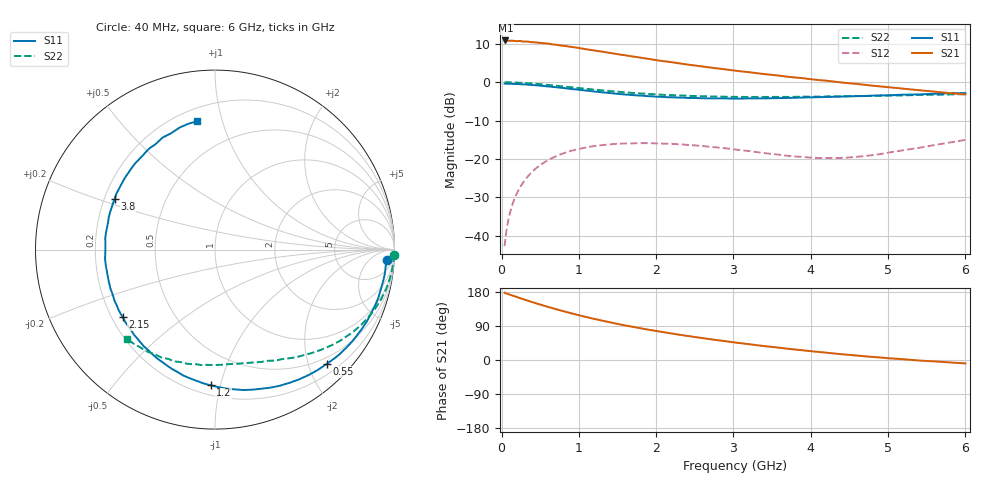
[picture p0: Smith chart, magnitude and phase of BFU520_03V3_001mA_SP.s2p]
! Filename:  P:\Prog\Test\Noise\ATS_data\Testdata_Net\03 Spar\BFU520_APG2013_37_A05_03p3V_001mA_SP_CM01_D.s2p
! Date/Time: Fri 26/Apr/2013 13:00:02
! BFU520_APG2013_37_A05_03p3V_1to20mA_SP_CM01_Bias1_R.s2p
! MDIF S-parameter v. bias file
! BFU520_APG2013_37_A05_03p3V_1to20mA_SP_CM01
! Date/time Tue Apr 23 14:11:50 2013
! bias mode 1
! bias variable = I_out
! VAR bias_var= 1
! VAR V_out= 3.3000
! VAR I_out= 0.9950
! VAR V_in= 0.7915
! VAR I_in= 0.0112
! Device data file deembeded for feedlines and parallel
! Original file: \03 Spar\BFU520_APG2013_37_A05_03p3V_001mA_SP_CM01_R.s2p
! Feed-files: PR047V01_250413_Feed1.s2p, PR047V01_250413_Feed2.s2p
! Parallel-file: PR047V01_250413_Par.s2p
# MHz S MA R 50
!  Freq-MHz  S11-mag  S11-arg  S21-mag  S21-arg  S12-mag  S12-arg  S22-mag  S22-arg
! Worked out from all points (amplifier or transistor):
!   98 points, 40 MHz to 6 GHz, reference 50 ohm
!   highest |S21| = 10.9 dB at 50 MHz (marker M1)
!   |S21| within 3 dB of that: start of sweep to 1.326 GHz
!   unconditionally stable (mu >= 1): 3.493 GHz to 5.423 GHz
!   at 300 MHz: K = 0.08, MSG = 18.1 dB, |S12| = -25.6 dB
!   at 1.6 GHz: K = 0.39, MSG = 11.5 dB, |S12| = -16.0 dB
!   at 6 GHz: K = 0.86, MSG = 5.9 dB, |S12| = -15.0 dB
!   S11 on the Smith chart (normalised r, x): 40 MHz: 16, -22; 550 MHz: 0.38, -2.32; 1.2 GHz: 0.26, -0.93; 2.15 GHz: 0.24, -0.31; 3.8 GHz: 0.24, +0.23; 6 GHz: 0.28, +0.83
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40  0.9581 -3.4  3.498 177.5  0.007263 87.4  0.9973 -1.7
50  0.9573 -4.2  3.506 176.0  0.009029 87.4  0.9976 -2.1
100  0.9555 -8.4  3.458 173.1  0.0181 84.3  0.9951 -4.5
120  0.9539 -10.2  3.488 171.6  0.02165 83.2  0.9937 -5.5
200  0.9485 -16.8  3.43 166.1  0.03576 78.6  0.9875 -9.2
240  0.9424 -20.4  3.448 163.2  0.04257 76.4  0.9838 -11.0
340  0.9295 -28.6  3.385 156.6  0.05896 71.0  0.9692 -15.5
550  0.8906 -45.7  3.224 143.2  0.08947 60.2  0.9315 -24.1
700  0.861 -57.2  3.091 134.4  0.1076 53.2  0.9011 -29.8
800  0.8401 -64.5  2.99 128.8  0.118 49.0  0.8792 -33.2
1050  0.7865 -82.0  2.742 115.6  0.1381 39.2  0.828 -41.1
1200  0.7568 -91.8  2.599 108.4  0.1466 33.9  0.8 -45.2
1600  0.6908 -115.7  2.245 91.2  0.1587 22.1  0.7373 -55.0
1850  0.6623 -129.0  2.052 81.8  0.1607 16.2  0.7094 -60.1
2050  0.6453 -138.8  1.91 75.0  0.1584 12.2  0.6882 -64.1
2150  0.6366 -144.0  1.851 71.5  0.1578 10.3  0.6806 -66.0
2600  0.6179 -163.5  1.603 57.8  0.1469 4.0  0.656 -74.3
3100  0.6115 176.8  1.385 44.2  0.1296 1.1  0.6432 -82.9
3800  0.6272 153.0  1.152 27.6  0.1076 6.6  0.6446 -95.1
4100  0.6378 143.8  1.067 21.3  0.1027 12.7  0.6484 -100.4
5200  0.6892 115.0  0.8229 2.0  0.1296 35.4  0.673 -120.1
6000  0.7218 98.1  0.6931 -9.0  0.1768 38.5  0.698 -134.6
